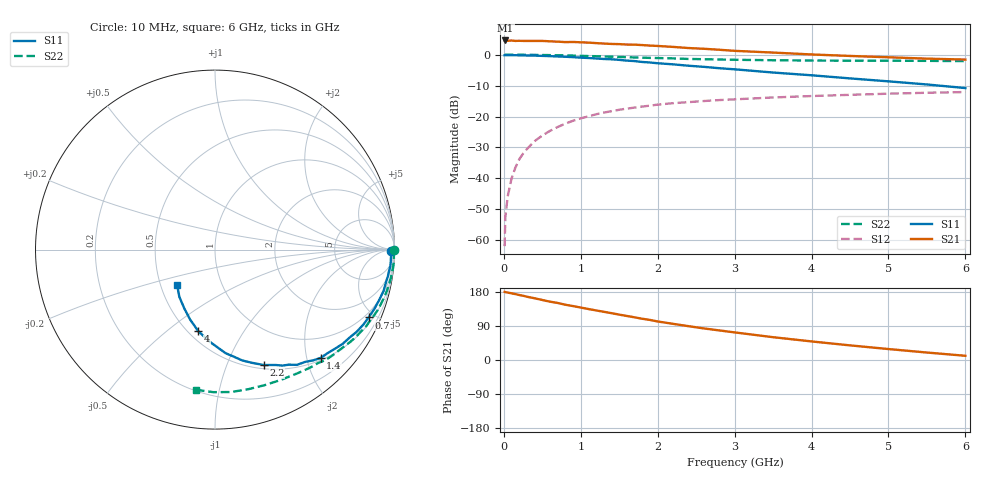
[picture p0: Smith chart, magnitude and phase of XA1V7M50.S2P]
! SIEMENS Discrete & RF Semiconductors
! BFY180
! Si NPN RF Bipolar Junction Transistor in MICRO-X
! VCE = 1.75 V  IC = 0.5 mA
! Common Emitter S-Parameters:  May  1997
# GHz  S  MA  R  50
!  f  S11  S21  S12  S22
! GHz  MAG  ANG  MAG  ANG  MAG  ANG  MAG  ANG
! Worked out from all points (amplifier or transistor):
!   36 points, 10 MHz to 6 GHz, reference 50 ohm
!   highest |S21| = 4.6 dB at 20 MHz (marker M1)
!   |S21| within 3 dB of that: start of sweep to 2.796 GHz
!   unconditionally stable (mu >= 1): 5.13 GHz to end of sweep
!   at 250 MHz: K = 0.05, MSG = 18.2 dB, |S12| = -32.0 dB
!   at 1.4 GHz: K = 0.41, MSG = 10.9 dB, |S12| = -18.3 dB
!   at 6 GHz: K = 1.04, MAG = 4.1 dB, |S12| = -12.1 dB
!   S11 on the Smith chart (normalised r, x): 10 MHz: 93, -24; 700 MHz: 0.76, -4.63; 1.4 GHz: 0.54, -2.26; 2.2 GHz: 0.54, -1.36; 4 GHz: 0.56, -0.65; 6 GHz: 0.61, -0.26
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0.01  0.98 -0.3  1.684 179.8  0.0008 93.0  0.9995 -0.2
0.02  0.9798 -0.8  1.699 179.0  0.0024 92.3  0.9999 -0.4
0.05  0.9816 -1.6  1.679 178.1  0.0051 89.1  0.9987 -1.1
0.1  0.9814 -3.4  1.696 175.9  0.0099 87.5  0.9973 -2.4
0.15  0.9815 -5.2  1.67 173.9  0.0149 86.2  0.9994 -3.5
0.2  0.9771 -6.8  1.678 171.5  0.0203 84.8  0.9976 -4.7
0.4  0.9672 -13.7  1.668 162.9  0.04 79.9  0.9929 -9.2
0.6  0.9479 -20.2  1.645 153.9  0.0586 74.3  0.9844 -13.8
0.7  0.936 -23.8  1.625 150.5  0.0678 71.4  0.9786 -16.0
0.8  0.9263 -26.8  1.598 145.8  0.0767 69.1  0.9728 -18.3
0.9  0.9122 -30.2  1.606 142.3  0.0855 66.5  0.9667 -20.4
1.1  0.8839 -36.5  1.567 134.5  0.1009 61.6  0.9502 -24.6
1.4  0.8432 -45.7  1.492 123.6  0.122 54.8  0.9268 -30.8
1.7  0.7879 -54.6  1.455 112.6  0.1395 48.8  0.901 -36.3
2.2  0.6981 -67.1  1.336 95.4  0.1644 40.0  0.8712 -44.9
2.6  0.6359 -76.2  1.246 83.3  0.178 34.2  0.8452 -50.9
2.8  0.6045 -80.2  1.202 78.1  0.1845 31.6  0.8355 -53.8
3.5  0.5145 -93.2  1.082 60.2  0.2033 23.5  0.8135 -63.2
4  0.4645 -101.5  1.009 49.0  0.2144 18.2  0.8043 -69.9
4.5  0.4136 -109.6  0.954 38.6  0.2243 13.5  0.7995 -76.7
5.5  0.33 -127.0  0.863 19.7  0.2423 4.3  0.7943 -90.7
6  0.2884 -137.1  0.834 11.1  0.2488 -0.4  0.7881 -97.7
